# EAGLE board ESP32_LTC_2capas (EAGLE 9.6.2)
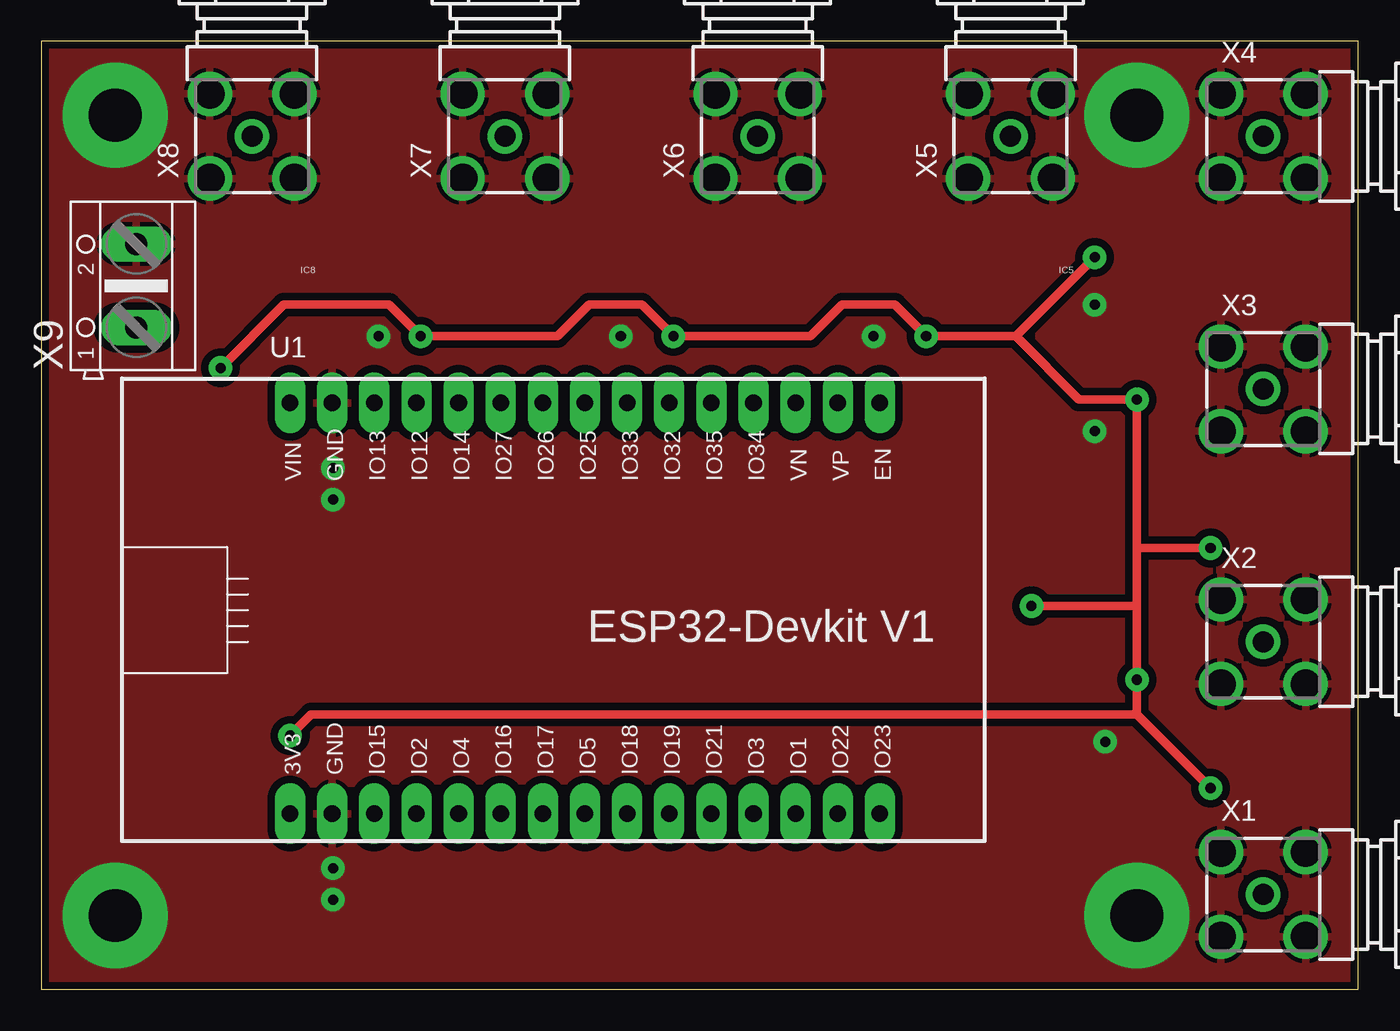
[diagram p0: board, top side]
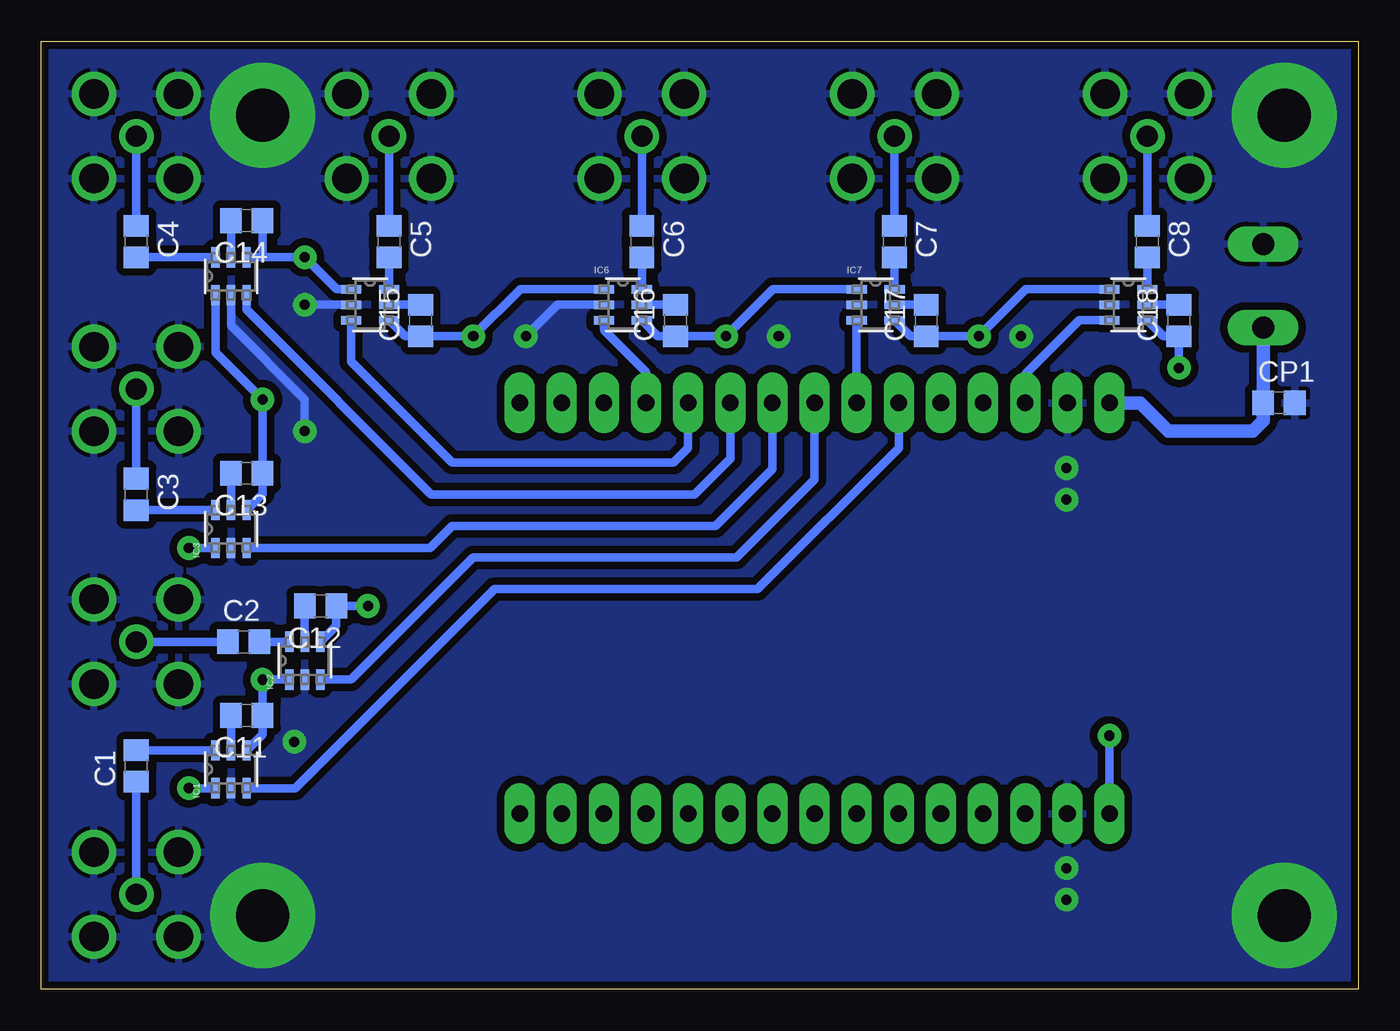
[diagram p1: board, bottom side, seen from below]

Size 79.38 x 57.15 mm. Coordinates in mm from the lower left corner, seen from the top.
Outline: 0,0 79.38,0 79.38,57.15 0,57.15 0,0
Copper layers (1*16): Top 0.035mm / dielectric 1.5mm / Bottom 0.035mm
Design rules "default *": minimum track width 6mil, minimum drill 0.35mm, track to track 6mil, track to pad 6mil, pad to pad 6mil, via to via 6mil, smd to smd 6mil, copper to edge 16mil, drill to drill 6mil, minimum pad ring 16mil, minimum via ring 12mil, stop-mask expansion 4mil, vias tented up to drill 0mil, thermal gap 10mil

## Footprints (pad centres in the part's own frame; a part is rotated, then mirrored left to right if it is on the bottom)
RCL_C0805 = smd 1.3 x 1.5: 1 -0.95,0; 2 0.95,0
SOT-23_S6 = smd 1.219 x 0.508: 1 -1.143,0.94; 2 -1.143,0; 3 -1.143,-0.94; 4 1.143,-0.94; 5 1.143,0; 6 1.143,0.94
ESP32-DEVKITV1_ESP32-DEVKITV1 = drill 1 pad 1.829 long: 1 -17.79,-11.635; 2 -15.25,-11.635; 3 -12.71,-11.635; 4 -10.17,-11.635; 5 -7.63,-11.635; 6 -5.09,-11.635; 7 -2.55,-11.635; 8 -0.01,-11.635; 9 2.53,-11.635; 10 5.07,-11.635; 11 7.61,-11.635; 12 10.15,-11.635; 13 12.69,-11.635; 14 15.23,-11.635; 15 17.77,-11.635; 16 17.77,13.135; 17 15.23,13.135; 18 12.69,13.135; 19 10.15,13.135; 20 7.61,13.135; 21 5.07,13.135; 22 2.53,13.135; 23 -0.01,13.135; 24 -2.55,13.135; 25 -5.09,13.135; 26 -7.63,13.135; 27 -10.17,13.135; 28 -12.71,13.135; 29 -15.25,13.135; 30 -17.79,13.135
BU-SMA-G = drill 1.27: 1 0,0 | drill 1.778: 2 -2.55,2.55; 3 2.55,2.55; 4 2.55,-2.55; 5 -2.55,-2.55
CGS_02_AK500/2 = drill 1.321 long: 1 -2.515,0; 2 2.515,0

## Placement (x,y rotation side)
C1  [RCL_C0805]  73.66,13.46 90 bottom
C2  [RCL_C0805]  67.18,20.96 0 bottom
C3  [RCL_C0805]  73.66,29.85 270 bottom
C4  [RCL_C0805]  73.66,45.08 270 bottom
C5  [RCL_C0805]  58.42,45.08 270 bottom
C6  [RCL_C0805]  43.18,45.08 270 bottom
C7  [RCL_C0805]  27.94,45.08 270 bottom
C8  [RCL_C0805]  12.7,45.08 270 bottom
C11  [RCL_C0805]  67,16.51 180 bottom
C12  [RCL_C0805]  62.55,23.11 180 bottom
C13  [RCL_C0805]  67,31.11 180 bottom
C14  [RCL_C0805]  67,46.36 180 bottom
C15  [RCL_C0805]  56.52,40.33 90 bottom
C16  [RCL_C0805]  41.15,40.33 90 bottom
C17  [RCL_C0805]  26.04,40.33 90 bottom
C18  [RCL_C0805]  10.79,40.33 90 bottom
CP1  [RCL_C0805]  4.76,35.36 0 bottom
IC1  LTC5507ES6TRMPBF  [SOT-23_S6]  67.94,13.27 90 bottom
IC2  LTC5507ES6TRMPBF  [SOT-23_S6]  63.5,19.81 90 bottom
IC3  LTC5507ES6TRMPBF  [SOT-23_S6]  67.94,27.75 90 bottom
IC4  LTC5507ES6TRMPBF  [SOT-23_S6]  67.94,42.99 90 bottom
IC5  LTC5507ES6TRMPBF  [SOT-23_S6]  59.56,41.28 0 bottom
IC6  LTC5507ES6TRMPBF  [SOT-23_S6]  44.32,41.28 0 bottom
IC7  LTC5507ES6TRMPBF  [SOT-23_S6]  29.08,41.28 0 bottom
IC8  LTC5507ES6TRMPBF  [SOT-23_S6]  13.84,41.28 0 bottom
U1  ESP32-DEVKITV1_ESP32DEVKITV1  [ESP32-DEVKITV1_ESP32-DEVKITV1]  32.78,22.23 0 top
X1  BU-SMA-G  [BU-SMA-G]  73.66,5.71 0 top
X2  BU-SMA-G  [BU-SMA-G]  73.66,20.96 0 top
X3  BU-SMA-G  [BU-SMA-G]  73.66,36.19 0 top
X4  BU-SMA-G  [BU-SMA-G]  73.66,51.44 0 top
X5  BU-SMA-G  [BU-SMA-G]  58.42,51.44 90 top
X6  BU-SMA-G  [BU-SMA-G]  43.18,51.44 90 top
X7  BU-SMA-G  [BU-SMA-G]  27.94,51.44 90 top
X8  BU-SMA-G  [BU-SMA-G]  12.7,51.44 90 top
X9  [CGS_02_AK500/2]  5.71,42.42 90 top

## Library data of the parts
C1-C8 C11-C18 CP1 = RDS_SasPe; SPICEPREFIX: C
IC1-IC8 = LTC5507ES6TRMPBF; AVAILABILITY: In Stock; CHECK_PRICES: https://www.snapeda.com/parts/LTC5507ES6%23TRMPBF/Analog+Devices/view-part/?ref=eda; DESCRIPTION: 100kHz to 1GHz RF Power Detector; MF: Analog Devices; MP: LTC5507ES6#TRMPBF; PACKAGE: SOT-6 Analog Devices; PRICE: None; PURCHASE-URL: https://www.snapeda.com/api/url_track_click_mouser/?unipart_id=4331394&manufacturer=Analog Devices&part_name=LTC5507ES6#TRMPBF&search_term=None; SNAPEDA_LINK: https://www.snapeda.com/parts/LTC5507ES6%23TRMPBF/Analog+Devices/view-part/?ref=snap
U1 = RDS_SasPe
X1-X8 = con-coax; OC_FARNELL: unknown; OC_NEWARK: unknown
X9 = CR30_2020_C

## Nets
3.3V: C11.1 C12.1 C13.1 C14.1 C15.1 C16.1 C17.1 C18.1 IC1.1 IC1.4 IC2.1 IC2.4 IC3.1 IC3.4 IC4.1 IC4.4 IC5.1 IC5.4 IC6.1 IC6.4 IC7.1 IC7.4 IC8.1 IC8.4 U1.1
GND: CP1.2 IC1.2 IC2.2 IC3.2 IC4.2 IC5.2 IC6.2 IC7.2 IC8.2 U1.2 U1.29 X1.2 X1.3 X1.4 X1.5 X2.2 X2.3 X2.4 X2.5 X3.2 X3.3 X3.4 X3.5 X4.2 X4.3 X4.4 X4.5 X5.2 X5.3 X5.4 X5.5 X6.2 X6.3 X6.4 X6.5 X7.2 X7.3 X7.4 X7.5 X8.2 X8.3 X8.4 X8.5 X9.2
N$1: C11.2 IC1.5
N$2: C1.2 IC1.6
N$3: C1.1 X1.1
N$4: C12.2 IC2.5
N$5: C2.2 IC2.6
N$6: C2.1 X2.1
N$7: C13.2 IC3.5
N$8: C3.2 IC3.6
N$9: C3.1 X3.1
N$10: C14.2 IC4.5
N$11: C4.2 IC4.6
N$12: C4.1 X4.1
N$13: C15.2 IC5.5
N$14: C5.2 IC5.6
N$15: C5.1 X5.1
N$16: C16.2 IC6.5
N$17: C6.2 IC6.6
N$18: C6.1 X6.1
N$19: C17.2 IC7.5
N$20: C7.2 IC7.6
N$21: C7.1 X7.1
N$22: C18.2 IC8.5
N$23: C8.2 IC8.6
N$24: C8.1 X8.1
SEN1: IC1.3 U1.25
SEN2: IC2.3 U1.23
SEN3: IC3.3 U1.22
SEN4: IC4.3 U1.21
SEN5: IC5.3 U1.20
SEN6: IC6.3 U1.19
SEN7: IC7.3 U1.24
SEN8: IC8.3 U1.28
VIN: CP1.1 U1.30 X9.1

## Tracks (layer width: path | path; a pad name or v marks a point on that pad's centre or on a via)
3.3V  (via drill 0.61 pad 1.42)
  Top 0.508: v63.5,44.14 58.74,39.38 | 58.74,39.38 v53.34,39.38 51.44,41.28 48.26,41.28 46.36,39.38 v38.1,39.38 36.2,41.28 33.02,41.28 31.12,39.38 v22.86,39.38 20.96,41.28 14.61,41.28 v10.79,37.47 | 58.74,39.38 62.55,35.56 v66.05,35.56 v66.04,35.56 66.04,26.67 66.05,26.67 66.05,26.61 | 66.05,23.11 v66.05,18.67 66.05,16.57 | 66.05,23.11 66.05,26.61 | v59.69,23.11 66.05,23.11 | v70.48,12.13 66.05,16.57 | 66.05,16.57 16.26,16.57 v14.99,15.3 | 66.05,26.61 v70.48,26.61
  Bottom 0.508: v10.79,37.47 C18.1 11.74,39.38 IC8.4 | IC7.4 26.98,39.38 C17.1 v22.86,39.38 20.02,42.22 IC8.1 | IC6.4 42.22,39.38 C16.1 v38.1,39.38 35.26,42.22 IC7.1 | IC3.4 66.05,29.86 C13.1 v66.05,35.56 68.89,38.4 IC4.1 | IC2.4 61.59,21.92 C12.1 v59.69,23.11 | IC1.4 66.05,15.37 C11.1 v66.05,18.67 IC2.1 | IC6.1 50.5,42.22 v53.34,39.38 C15.1 57.46,39.38 IC5.4 | C14.1 66.05,44.14 | 66.05,44.14 IC4.4 | 66.05,44.14 v63.5,44.14 61.58,42.22 IC5.1 | IC3.1 v70.48,26.61 | v70.48,12.13 IC1.1 | U1.1 v14.99,15.3
GND  (via drill 0.61 pad 1.42, 3.17 pad 6.35)
  Bottom 0.508: IC5.2 v63.5,41.28 | IC4.2 67.94,40 63.5,35.56 v63.5,33.66 | v50.16,39.38 48.27,41.28 IC6.2
  other vias: 4.45,52.7 66.04,52.7 4.45,4.45 66.04,4.45 34.92,39.38 20.32,39.38 64.14,14.92 17.58,7.3 17.58,5.4 17.58,31.43 17.58,29.53
  pour Top (isolate 0.457): -1.27,-5.71 -1.27,70.48 1.27,71.75 88.9,71.75 90.17,70.48 90.17,-4.45 88.9,-5.71
  pour Bottom (isolate 0.457): -0.64,71.75 90.81,71.75 90.81,-6.35 1.27,-6.35 -0.64,-4.45
N$1
  Bottom 0.508: IC1.5 C11.2
N$2
  Bottom 0.508: C1.2 IC1.6
N$3
  Bottom 0.508: X1.1 C1.1
N$4
  Bottom 0.508: IC2.5 C12.2
N$5
  Bottom 0.508: IC2.6 C2.2
N$6
  Bottom 0.508: C2.1 X2.1
N$7
  Bottom 0.508: IC3.5 C13.2
N$8
  Bottom 0.508: IC3.6 C3.2
N$9
  Bottom 0.508: C3.1 X3.1
N$10
  Bottom 0.508: IC4.5 C14.2
N$11
  Bottom 0.508: C4.2 IC4.6
N$12
  Bottom 0.508: C4.1 X4.1
N$13
  Bottom 0.508: IC5.5 C15.2
N$14
  Bottom 0.508: IC5.6 C5.2
N$15
  Bottom 0.508: C5.1 X5.1
N$16
  Bottom 0.508: IC6.5 C16.2
N$17
  Bottom 0.508: IC6.6 C6.2
N$18
  Bottom 0.508: C6.1 X6.1
N$19
  Bottom 0.508: IC7.5 C17.2
N$20
  Bottom 0.508: IC7.6 C7.2
N$21
  Bottom 0.508: C7.1 X7.1
N$22
  Bottom 0.508: C18.2 IC8.5
N$23
  Bottom 0.508: IC8.6 C8.2
N$24
  Bottom 0.508: C8.1 X8.1
SEN1
  Bottom 0.508: U1.25 27.69,32.64 36.2,24.13 52.07,24.13 64.07,12.13 IC1.3
SEN2
  Bottom 0.508: IC2.3 60.71,18.67 53.34,26.04 37.47,26.04 32.77,30.73 U1.23
SEN3
  Bottom 0.508: IC3.3 55.94,26.61 54.61,27.94 38.73,27.94 35.31,31.37 U1.22
SEN4
  Bottom 0.508: IC4.3 67,40.97 55.88,29.85 40.01,29.85 37.85,32 U1.21
SEN5
  Bottom 0.508: IC5.3 60.71,37.85 54.61,31.75 41.27,31.75 40.39,32.64 U1.20
SEN6
  Bottom 0.508: U1.19 42.93,37.21 45.47,39.75 IC6.3
SEN7
  Bottom 0.508: U1.24 IC7.3
SEN8
  Bottom 0.508: IC8.3 16.82,40.33 20.07,37.08 U1.28
VIN
  Bottom 0.813: X9.1 CP1.1 5.71,34.29 6.35,33.66 11.43,33.66 13.13,35.36 U1.30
